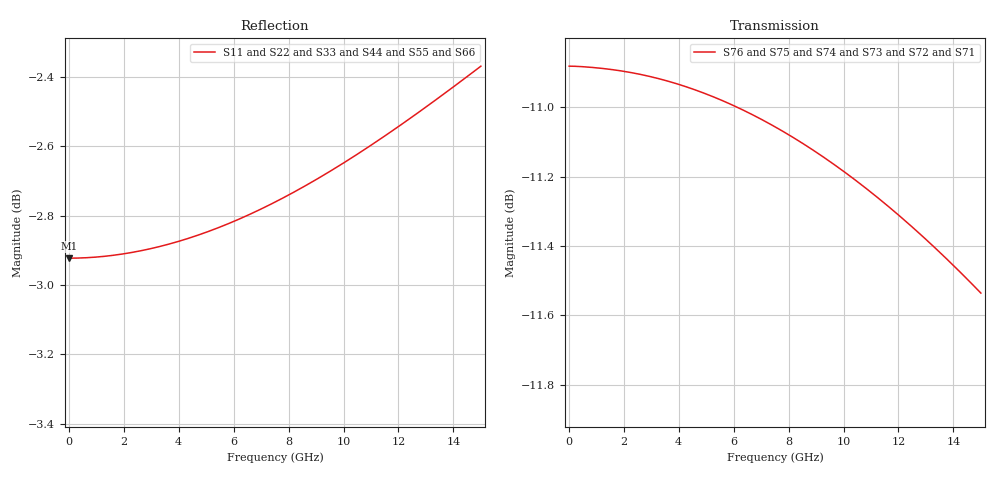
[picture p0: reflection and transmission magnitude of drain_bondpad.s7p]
! Created Wed Jan  6 11:14:07 2021
# hz S ma R 50
! 7 Port Network Data from SP1.SP block
! freq  magS11  angS11  magS12  angS12  magS13  angS13  magS14  angS14
!  magS15  angS15  magS16  angS16  magS17  angS17
!  magS21  angS21
!  magS22  angS22  magS23  angS23  magS24  angS24  magS25  angS25
!  magS26  angS26  magS27  angS27
!  magS31  angS31  magS32  angS32
!  magS33  angS33  magS34  angS34  magS35  angS35  magS36  angS36
!  magS37  angS37
!  magS41  angS41  magS42  angS42  magS43  angS43
!  magS44  angS44  magS45  angS45  magS46  angS46  magS47  angS47
!  magS51  angS51  magS52  angS52  magS53  angS53  magS54  angS54
!  magS55  angS55  magS56  angS56  magS57  angS57
!  magS61  angS61
!  magS62  angS62  magS63  angS63  magS64  angS64  magS65  angS65
!  magS66  angS66  magS67  angS67
!  magS71  angS71  magS72  angS72
!  magS73  angS73  magS74  angS74  magS75  angS75  magS76  angS76
!  magS77  angS77
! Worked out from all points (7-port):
!   1500 points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, 10 MHz to 15 GHz, reference 50 ohm
!   strongest paths, dB at 10 MHz, 3.76 GHz, 7.51 GHz, 11.26 GHz, 15 GHz:
!     S76: -10.9, -10.9, -11.1, -11.3, -11.5
!     S75: -10.9, -10.9, -11.1, -11.3, -11.5
!     S74: -10.9, -10.9, -11.1, -11.3, -11.5
!     S73: -10.9, -10.9, -11.1, -11.3, -11.5
!     S72: -10.9, -10.9, -11.1, -11.3, -11.5
!     S71: -10.9, -10.9, -11.1, -11.3, -11.5
!   lowest |S11| = -2.9 dB at 10 MHz (marker M1), VSWR 6.00, Z = 8.33 - j0.0026 ohm
!   |S11| at or under -10 dB: nowhere
